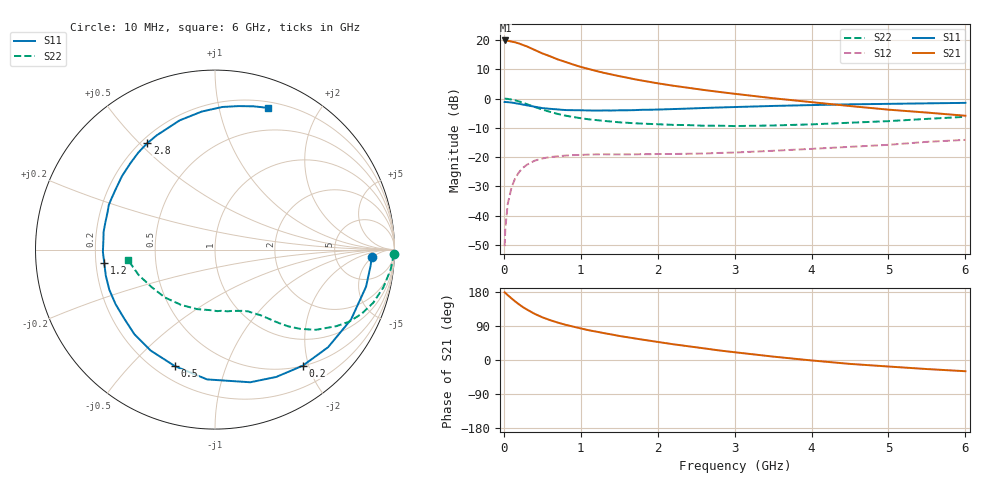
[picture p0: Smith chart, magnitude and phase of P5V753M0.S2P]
! SIEMENS Small Signal Semiconductors
! BFP183
! Si NPN RF Bipolar Junction Transistor in SOT143
! VCE = 0.75 V  IC = 3 mA
! Common Emitter S-Parameters:  March  1996
# GHz  S  MA  R  50
!  f  S11  S21  S12  S22
! GHz  MAG  ANG  MAG  ANG  MAG  ANG  MAG  ANG
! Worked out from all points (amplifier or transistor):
!   36 points, 10 MHz to 6 GHz, reference 50 ohm
!   highest |S21| = 19.8 dB at 20 MHz (marker M1)
!   |S21| within 3 dB of that: start of sweep to 380.2 MHz
!   unconditionally stable (mu >= 1): 1.757 GHz to end of sweep
!   at 250 MHz: K = 0.17, MSG = 21.0 dB, |S12| = -23.6 dB
!   at 1.4 GHz: K = 0.83, MSG = 13.7 dB, |S12| = -19.1 dB
!   at 6 GHz: K = 1.12, MAG = 2.0 dB, |S12| = -14.1 dB
!   S11 on the Smith chart (normalised r, x): 10 MHz: 13, -5; 200 MHz: 0.50, -1.90; 500 MHz: 0.28, -0.68; 1.2 GHz: 0.23, -0.06; 2.8 GHz: 0.23, +0.53; 6 GHz: 0.26, +1.41
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0.01  0.8738 -2.7  9.721 178.6  0.003 88.6  0.9948 -1.3
0.02  0.8717 -5.9  9.819 177.0  0.0061 84.2  0.9929 -2.6
0.05  0.8666 -13.8  9.704 171.2  0.0156 83.6  0.9849 -6.5
0.1  0.8522 -27.2  9.391 162.6  0.0303 74.5  0.9612 -12.7
0.15  0.8323 -40.8  9.113 154.1  0.0442 67.8  0.9299 -18.6
0.2  0.8109 -52.9  8.693 146.4  0.0557 61.7  0.8915 -23.7
0.25  0.7873 -64.3  8.192 139.3  0.0657 55.8  0.8479 -28.3
0.3  0.7648 -75.1  7.768 133.2  0.0739 51.0  0.8001 -32.2
0.4  0.7246 -93.5  6.763 121.9  0.0866 42.9  0.7181 -38.5
0.5  0.6865 -109.0  5.9 112.7  0.0946 36.4  0.6488 -42.9
0.6  0.6671 -122.4  5.278 105.2  0.0998 31.5  0.5918 -46.3
0.7  0.651 -133.7  4.661 98.8  0.103 27.8  0.5454 -48.8
0.8  0.6348 -143.2  4.223 93.0  0.1058 24.7  0.5103 -50.8
1.1  0.6254 -166.7  3.205 78.7  0.1101 18.7  0.442 -55.5
1.2  0.6215 -173.1  2.957 74.9  0.111 17.0  0.4284 -57.1
1.7  0.6335 161.0  2.134 57.0  0.1111 14.2  0.3779 -64.8
2.2  0.6604 141.7  1.656 41.6  0.1128 13.8  0.3546 -74.2
2.8  0.7027 122.5  1.296 25.2  0.1175 14.9  0.3431 -87.9
3.5  0.7467 105.2  1.011 9.0  0.1279 16.8  0.3463 -106.7
4.5  0.7956 87.1  0.744 -10.3  0.1494 16.3  0.3859 -136.3
5.5  0.8271 74.8  0.575 -23.9  0.1819 14.0  0.4487 -161.7
6  0.8425 69.6  0.508 -29.6  0.1966 10.5  0.4869 -173.0
